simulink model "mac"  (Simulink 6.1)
settings: Solver=ode45  StartTime=0.0  StopTime=20  RelTol=1e-3
undefined symbols (not defined in the file or in its folder): coef, Ft, netlist
libraries: xbsIndex_r3 x13

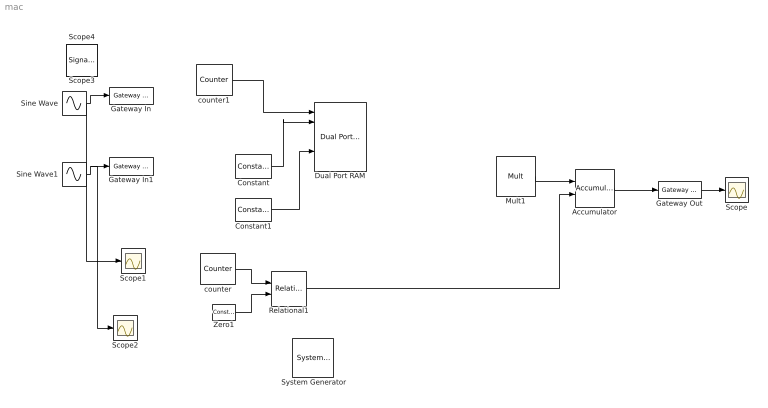
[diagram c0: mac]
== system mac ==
  " System Generator" : xbsIndex_r3/ System Generator  Tag=genX  xilinxfamily=Virtex2  part=xc2v1000  speed=-4  package=bg575  synthesis_tool=XST  directory=./netlist  testbench=off  simulink_period=1/2  sysclk_period=100  incr_netlist=off  trim_vbits=Everywhere in SubSystem  dbl_ovrd=According to Block Masks  core_generation=According to Block Masks  run_coregen=off  deprecated_control=off  eval_field=0
  Accumulator : xbsIndex_r3/Accumulator  n_bits=8  overflow=Wrap  operation=Add  scale=1  explicit_period=off  period=1  rst=on  hasbypass=off  en=off  dbl_ovrd=off  show_param=off  gen_core=off  use_rpm=on
  Constant : xbsIndex_r3/Constant  const=2  equ=P=C  arith_type=Unsigned  n_bits=2  bin_pt=0  opselect=C  inp2=PCIN>>17  opr=+  inp1=P  carry=CIN  iostate=0  explicit_period=on  period=1  dbl_ovrd=off
  Constant1 : xbsIndex_r3/Constant  const=3  equ=P=C  arith_type=Unsigned  n_bits=2  bin_pt=0  opselect=C  inp2=PCIN>>17  opr=+  inp1=P  carry=CIN  iostate=0  explicit_period=on  period=1  dbl_ovrd=off
  Dual Port RAM : xbsIndex_r3/Dual Port RAM  depth=16  initVector=sin(pi*(0:15)/16)  write_mode_A=Read After Write  write_mode_B=Read After Write  latency=1  mem_collision=off  init_zero=on  explicit_period=off  period=1  dbl_ovrd=off  rst_a=off  init_a=0  rst_b=off  init_b=0  show_param=off  distributed_mem=off  use_rpm=off  gen_core=off
  Gateway In : xbsIndex_r3/Gateway In  arith_type="Signed  (2's comp)"  n_bits=8  bin_pt=6  quantization=Truncate  overflow=Wrap  period=1  timing_constraint=None  locs_specified=off  LOCs={}  needs_fixed_name=off  dbl_ovrd=off  show_param=off
  Gateway In1 : xbsIndex_r3/Gateway In  arith_type="Signed  (2's comp)"  n_bits=8  bin_pt=6  quantization=Truncate  overflow=Wrap  period=1  timing_constraint=None  locs_specified=off  LOCs={}  needs_fixed_name=off  dbl_ovrd=off  show_param=off
  Gateway Out : xbsIndex_r3/Gateway Out  output_type=Double  nbits=8  bin_pt=6  arith_type=Boolean  quantization=Truncate  overflow=Wrap  hdl_port=on  timing_constraint=None  locs_specified=off  LOCs={}  needs_fixed_name=off  show_param=off
  Mult1 : xbsIndex_r3/Mult  precision=Full  arith_type="Signed  (2's comp)"  n_bits=8  bin_pt=2  quantization=Truncate  overflow=Wrap  latency=0  explicit_period=on  period=1  en=off  dbl_ovrd=off  show_param=off  mult_type=Parallel  oversample=2  use_embedded=off  pipeline=on  use_rpm=on  placement_style=Rectangular Shape  gen_core=off
  Relational1 : xbsIndex_r3/Relational  mode=a=b  latency=0  explicit_period=on  period=-1  en=off  dbl_ovrd=off  show_param=off
  Scope : Scope
  Scope1 : Scope
  Scope2 : Scope
  Sine Wave : Sin  Amplitude=.5  Frequency=2*pi/23  Phase=pi/6  SampleTime=1
  Sine Wave1 : Sin  Amplitude=.5  Frequency=2*pi/23  Phase=pi/6  SampleTime=1
  Zero1 : xbsIndex_r3/Constant  Priority=5  const=4  equ=P=C  arith_type=Unsigned  n_bits=3  bin_pt=0  opselect=C  inp2=PCIN>>17  opr=+  inp1=P  carry=CIN  iostate=0  explicit_period=off  period=Ft/length(coef)  dbl_ovrd=off
  counter : xbsIndex_r3/Counter  Priority=5  cnt_type=Count Limited  n_bits=3  bin_pt=0  arith_type=Unsigned  start_count=0  cnt_to=4  cnt_by_val=1  operation=Up  explicit_period=off  period=1  load_pin=off  rst=off  en=off  dbl_ovrd=off  show_param=off  use_rpm=on  gen_core=on
  counter1 : xbsIndex_r3/Counter  Priority=5  cnt_type=Count Limited  n_bits=3  bin_pt=0  arith_type=Unsigned  start_count=0  cnt_to=4  cnt_by_val=1  operation=Up  explicit_period=off  period=1  load_pin=off  rst=off  en=off  dbl_ovrd=off  show_param=off  use_rpm=on  gen_core=on
  Scope3 : SignalViewerScope  IOType=viewer  RefreshTime=0.035000
  Scope4 : SignalViewerScope  IOType=viewer  RefreshTime=0.035000
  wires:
  Gateway Out/1 -> Scope/1
  Sine Wave/1 -> Gateway In/1, Scope1/1
  Sine Wave1/1 -> Gateway In1/1, Scope2/1
  Mult1/1 -> Accumulator/1
  Accumulator/1 -> Gateway Out/1
  counter/1 -> Relational1/1
  Zero1/1 -> Relational1/2
  Relational1/1 -> Accumulator/2
  counter1/1 -> Dual Port RAM/1
  Constant/1 -> Dual Port RAM/2
  Constant1/1 -> Dual Port RAM/5
